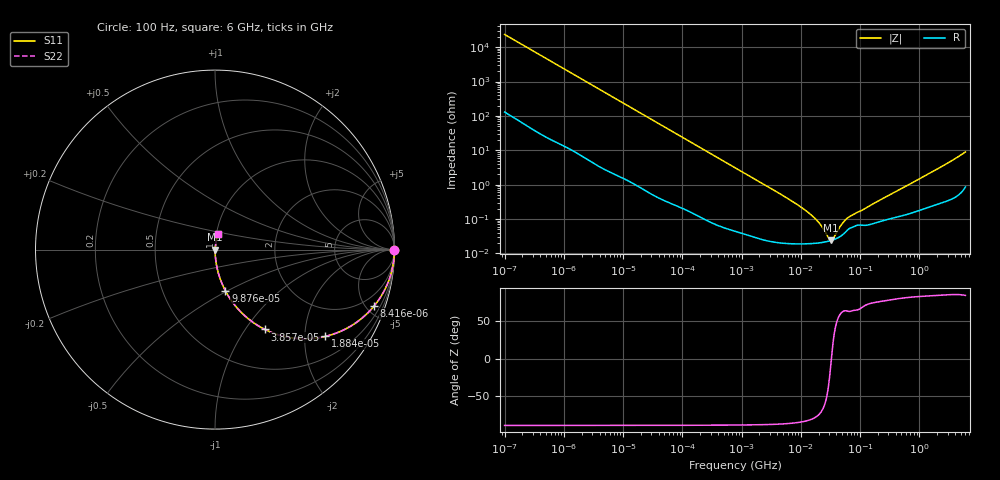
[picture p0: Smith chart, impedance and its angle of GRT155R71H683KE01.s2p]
!Murata Part Number: GRT155R71H683KE01
!These Parameters are Measured in Series Mode Connection
!Data Generated on Jun 19, 2026
!  o--ll--o
!Port1  Port2
!  o------o
!Operation Temp=25[degC], DC Bias Voltage=0[V]
!Freq. Start=100[Hz] Stop=6[GHz] 401[Steps]
# Hz S RI R 50
!Freq.(Hz) S11(Real) S11(Imag) S21(Real) S21(Imag) S12(Real) S12(Imag) S22(Real) S22(Imag)
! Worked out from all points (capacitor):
!   401 points, 100 Hz to 6 GHz, reference 50 ohm
!   read as one part in series: C = 67.9 nF near 109 Hz
!   lowest |Z| = 23.9 mohm at 31.85 MHz (marker M1)
!   series resonance near 32.85 MHz, so ESL is about 350 pH
!   S11 on the Smith chart (normalised r, x): 100 Hz: open; 8.416 kHz: 1.04, -5.65; 18.84 kHz: 1.02, -2.53; 38.57 kHz: 1.01, -1.24; 98.76 kHz: 1.00, -0.49; 6 GHz: 1.02, +0.18
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100  1 -0.00427  4.18e-05 0.00427  4.18e-05 0.00427  1 -0.00427
2008  0.9924 -0.0842  0.00764 0.0842  0.00764 0.0842  0.9924 -0.0842
4702  0.9612 -0.1904  0.0388 0.1904  0.0388 0.1904  0.9612 -0.1904
8416  0.887 -0.3135  0.113 0.3135  0.113 0.3135  0.887 -0.3135
18841  0.6149 -0.4833  0.3851 0.4833  0.3851 0.4833  0.6149 -0.4833
26957  0.4401 -0.4931  0.5599 0.4931  0.5599 0.4931  0.4401 -0.4931
38569  0.2789 -0.4451  0.7211 0.4451  0.7211 0.4451  0.2789 -0.4451
40335  0.2615 -0.436  0.7385 0.436  0.7385 0.436  0.2615 -0.436
60352  0.1379 -0.3411  0.8621 0.3411  0.8621 0.3411  0.1379 -0.3411
98762  0.0575 -0.2286  0.9425 0.2286  0.9425 0.2286  0.0575 -0.2286
241822  0.0108 -0.0986  0.9892 0.0986  0.9892 0.0986  0.0108 -0.0986
774597  0.00142 -0.0313  0.9986 0.0313  0.9986 0.0313  0.00142 -0.0313
6353432  0.000205 -0.00371  0.9998 0.00371  0.9998 0.00371  0.000205 -0.00371
1.555665e7  0.000194 -0.00122  0.9998 0.00122  0.9998 0.00122  0.000194 -0.00122
2.128304e7  0.000204 -0.000668  0.9998 0.000668  0.9998 0.000668  0.000204 -0.000668
2.911731e7  0.000225 -0.00018  0.9998 0.00018  0.9998 0.00018  0.000225 -0.00018
3.184506e7  0.000234 -4.62e-05  0.9998 4.62e-05  0.9998 4.62e-05  0.000234 -4.62e-05
3.482834e7  0.000246 8.78e-05  0.9998 -8.78e-05  0.9998 -8.78e-05  0.000246 8.78e-05
4.764863e7  0.00032 0.000571  0.9997 -0.000571  0.9997 -0.000571  0.00032 0.000571
6.233367e7  0.00049 0.000974  0.9995 -0.000974  0.9995 -0.000974  0.00049 0.000974
3.124326e8  0.00102 0.00484  0.999 -0.00484  0.999 -0.00484  0.00102 0.00484
6e9  0.0162 0.0869  0.9838 -0.0869  0.9838 -0.0869  0.0162 0.0869
